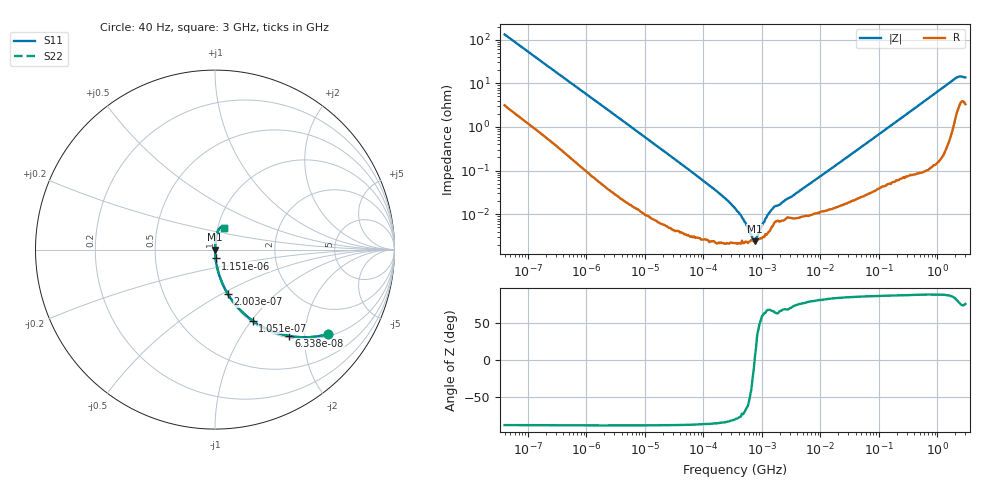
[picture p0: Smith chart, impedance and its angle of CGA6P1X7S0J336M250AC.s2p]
! S-parameter Generated by TDK Corporation
! Copyright(C) 2015 TDK Corporation.
! All Rights Reserved.
! TDK P/N: CGA6P1X7S0J336M250AC (Multilayer Ceramic Chip Capacitors)
! Property: C=33uF
! Size(LxWxT): 3.2x2.5x2.5mm, 0.126x0.098x0.098inches
! Model Type: s2p (Touchstone File Format Version 1.0)
! Frequency: DC=Yes Start=0.00004MHz Stop=3000MHz 396points Log-sweep
! Note: This model was converted from impedance.
! Model Generated on Jun. 23, 2015
! Hash(MD5):
! Port Assignments:
!  1 ---| |--- 2
! Applicable Conditions:
!  Temperature = 25 degC
!  DC Bias Voltage = 0 V
!  Small Signal Operation
! Terms and conditions regarding TDK Simulation Models
! (1)This simulation model is being provided solely for informational purposes. Please refer to the specifications of the products in terms of detailed characteristics of such products.
! (2)In no event shall TDK Corporation of any of its subsidiaries be liable for any loss or damage arising, directly or indirectly,
!  From any information contained in this simulation model, including, but not limited to loss or damages arising from any inaccuracies, omissions or errors in connection with such information.
! (3)Any and all copyrights on this simulation model are owned by TDK Corporation.
!  Duplication or redistribution of this simulation model without prior written permission from TDK Corporation is prohibited.
! (4)This simulation model is subject to any modification or change without any prior notice.
! (5)Neither TDK Corporation nor any of its subsidiaries shall make any warranty, express or implied,
!  Including but not limited to the correctness, implied warranties of merchantability and fitness for a particular purpose with respect to this simulation models.
! (6)The use of this simulation model shall be deemed to have consented to the terms and conditions hereof.
# MHz S MA R 50
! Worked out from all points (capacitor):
!   395 points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, 40 Hz to 3 GHz, reference 50 ohm
!   read as one part in series: C = 30.2 uF near 41.88 Hz
!   lowest |Z| = 2.42 mohm at 757.5 kHz (marker M1)
!   series resonance near 750.1 kHz, so ESL is about 1.5 nH
!   S11 on the Smith chart (normalised r, x): 40 Hz: 1.06, -2.63; 63.38 Hz: 1.04, -1.67; 105.1 Hz: 1.02, -1.01; 200.3 Hz: 1.01, -0.54; 1.151 kHz: 1.00, -0.10; 3 GHz: 1.07, +0.26
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4e-05  0.7868 -36.8  0.5987 51.9  0.5987 51.9  0.7868 -36.8
6.337743e-05  0.6338 -49.4  0.759 39.3  0.759 39.3  0.6338 -49.4
0.000105147  0.4482 -62.1  0.8838 26.6  0.8838 26.6  0.4482 -62.1
0.0002002725  0.2591 -73.7  0.9603 15.0  0.9603 15.0  0.2591 -73.7
0.0003814572  0.1423 -80.7  0.987 8.2  0.987 8.2  0.1423 -80.7
0.000834128  0.06716 -85.2  0.9966 3.9  0.9966 3.9  0.06716 -85.2
0.001151185  0.04913 -86.2  0.998 2.8  0.998 2.8  0.04913 -86.2
0.01739424  0.00338 -88.7  0.9999 0.2  0.9999 0.2  0.00338 -88.7
0.1317813  0.0004429 -86.9  1 0.0  1 0.0  0.0004429 -86.9
0.2397126  0.0002274 -84.7  1 0.0  1 0.0  0.0002274 -84.7
0.3464102  0.000137 -80.9  1 0.0  1 0.0  0.000137 -80.9
0.4164285  0.0001013 -77.7  1 0.0  1 0.0  0.0001013 -77.7
0.7574911  2.421e-05 3.6  1 -0.0  1 -0.0  2.421e-05 3.6
1.256723  9.799e-05 67.8  1 -0.0  1 -0.0  9.799e-05 67.8
1.656397  0.0001521 64.3  0.9999 -0.0  0.9999 -0.0  0.0001521 64.3
1.991197  0.000165 65.8  0.9999 -0.0  0.9999 -0.0  0.000165 65.8
7.22376  0.0005464 79.6  0.9999 -0.0  0.9999 -0.0  0.0005464 79.6
150.6385  0.01016 86.6  0.9994 -0.6  0.9994 -0.6  0.01016 86.6
687.8953  0.04465 86.1  0.998 -2.6  0.998 -2.6  0.04465 86.1
1982.595  0.1253 76.6  0.9787 -7.2  0.9787 -7.2  0.1253 76.6
2383.329  0.1378 69.6  0.9606 -7.7  0.9606 -7.7  0.1378 69.6
3000  0.131 68.6  0.96 -7.3  0.96 -7.3  0.131 68.6
